(* Logix 5000 AddOnInstructionDefinition export Banner_Q4X_Teach_v4; software revision 36.00 *)

TYPE Banner_IOL_Port_v4 :   // UDT that has all of the data items necessary to communicate with a specific Port on a IO-Link Master
STRUCT
   Port_Controlled : INT;   // Each bit represents a port on an IO-Link Master. Set to 1 to tell AOI to control that port.
   Port_Activate : INT;   // Each bit represents a port on an IO-Link Master. When ON that port will process any commands in queue.
   Port_Read : INT;   // Each bit represents a port on an IO-Link Master. Used to determine when device AOI has requested a Read command.
   Port_Write : INT;   // Each bit represents a port on an IO-Link Master. Used to determine when device AOI has requested a Write command.
   Port_RW_Complete : INT;   // Each bit represents a port on an IO-Link Master. Tells device AOI that Read or Write request has been completed.
   Port_Device_Read : INT;
   Data_Transfer : SINT[190];   // Array to transfer data from IO-Master to device AOIs.
END_STRUCT
END_TYPE

TYPE Banner_Q4X_Data_v4 :   // UDT that stores Teach Data for a Q4X.
STRUCT
   System_Command : INT;   // Write Only. See IODD file for list of commands that can be activated via the System Command interface
   Teach_Channel : INT;   // RW. 0 = Default, 1 = BDC1, 2 = BDC2
   Teach_State : SINT;   // Read Only. 0 =IDLE, 1 = SP1 Success, 4 = Wait for Command, 5 = Busy, 7 = Error
   SP1_TP1 : SINT;   // Read Only. 0 = not taught or unsuccessful, 1 = successfully taught
   SP2_TP2 : SINT;   // Read Only. 0 = not taught or unsuccessful, 1 = successfully taught
   BDC1_Setpoint_SP1 : DINT;   // Switch point value in .1 mm increments. Range: varies depending on sensor.
   BDC1_Setpoint_SP2 : DINT;   // In FGS mode defines second switching point parameter. Range: varies depending on sensor.
   BDC2_Setpoint_SP1 : DINT;   // Switch point value in .1 mm increments. Range: varies depending on sensor.
   BDC2_Setpoint_SP2 : DINT;   // In FGS mode defines second switching point parameter. Range: varies depending on sensor.
END_STRUCT
END_TYPE

TYPE Banner_Q4X_v4 :   // All of the parameters for a Q4X.
STRUCT
   Initial_Global_Read : BOOL;   // Determines if all of the IO-Link data has been read into the PLC yet
   Command : INT;   // Value placed in here will activate a read or write to a specifc IO-Link Index
   Data : Banner_Q4X_Data_v4;   // Write Data
   Reset : BOOL;   // Resets AOI. This will force a complete parameter read of the sensor.
END_STRUCT
END_TYPE

ADD_ON_INSTRUCTION Banner_Q4X_Teach_v4   (* revision 4.2, vendor Banner Engineering *)
// AOI to read and write parameter data to an IO-Link Q4X.
// Revision note:
// AOI to only access Standard Command IO-Link function. This is used to teach the sensor. It also accesses the Teach Status.
VAR_IN_OUT
   Q4X : Banner_Q4X_v4; {required}
   Port_Data : Banner_IOL_Port_v4; {required}
END_VAR
VAR_INPUT
   Port : INT; {required}   // Enter the Port number that this AOI is to work with.
END_VAR
VAR_IN_OUT
   Teach : BOOL; {required}
END_VAR
VAR_OUTPUT
   Teach_Error : BOOL; {visible}
END_VAR
VAR
   Local_Control : DINT; {access None}
   Global_Read_Command_Value : INT; {access None}
   Global_Write_Command_Value : INT; {access None}
   Command_Being_Processed : BOOL; {access None}
   Update_Archive : BOOL; {access None}
   Index_Write_Inprocess : INT; {access None}
   Index_Write_Control : INT; {access None}
   Temp_Excess_Gain : DINT[2]; {access None}
   Inprocess_Index : DINT; {access None}
   Counter : COUNTER := (PRE := 20); {access None}
   WriteCheck : BOOL; {access None}
   Timer2 : TIMER := (PRE := 7500); {access None}
   Timer1 : TIMER := (PRE := 60000); {access None}
END_VAR

ROUTINE Logic   (* ladder *)
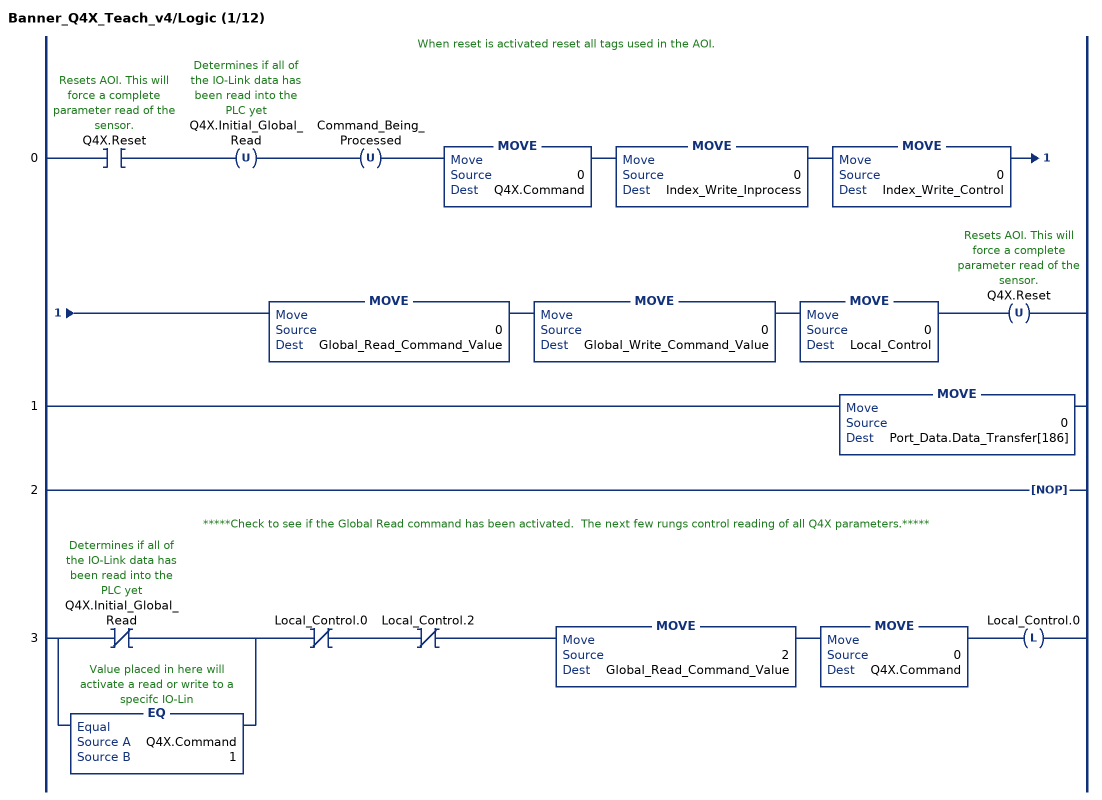
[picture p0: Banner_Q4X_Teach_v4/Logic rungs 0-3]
   // When reset is activated reset all tags used in the AOI.
   0: XIC(Q4X.Reset)OTU(Q4X.Initial_Global_Read)OTU(Command_Being_Processed)MOVE(0,Q4X.Command)MOVE(0,Index_Write_Inprocess)MOVE(0,Index_Write_Control)MOVE(0,Global_Read_Command_Value)MOVE(0,Global_Write_Command_Value)MOVE(0,Local_Control)OTU(Q4X.Reset);
   1: MOVE(0,Port_Data.Data_Transfer[186]);
   2: NOP();
   // *****Check to see if the Global Read command has been activated.  The next few rungs control reading of all Q4X parameters.*****
   3: [XIO(Q4X.Initial_Global_Read) ,EQ(Q4X.Command,1) ]XIO(Local_Control.0)XIO(Local_Control.2)MOVE(2,Global_Read_Command_Value)MOVE(0,Q4X.Command)OTL(Local_Control.0);
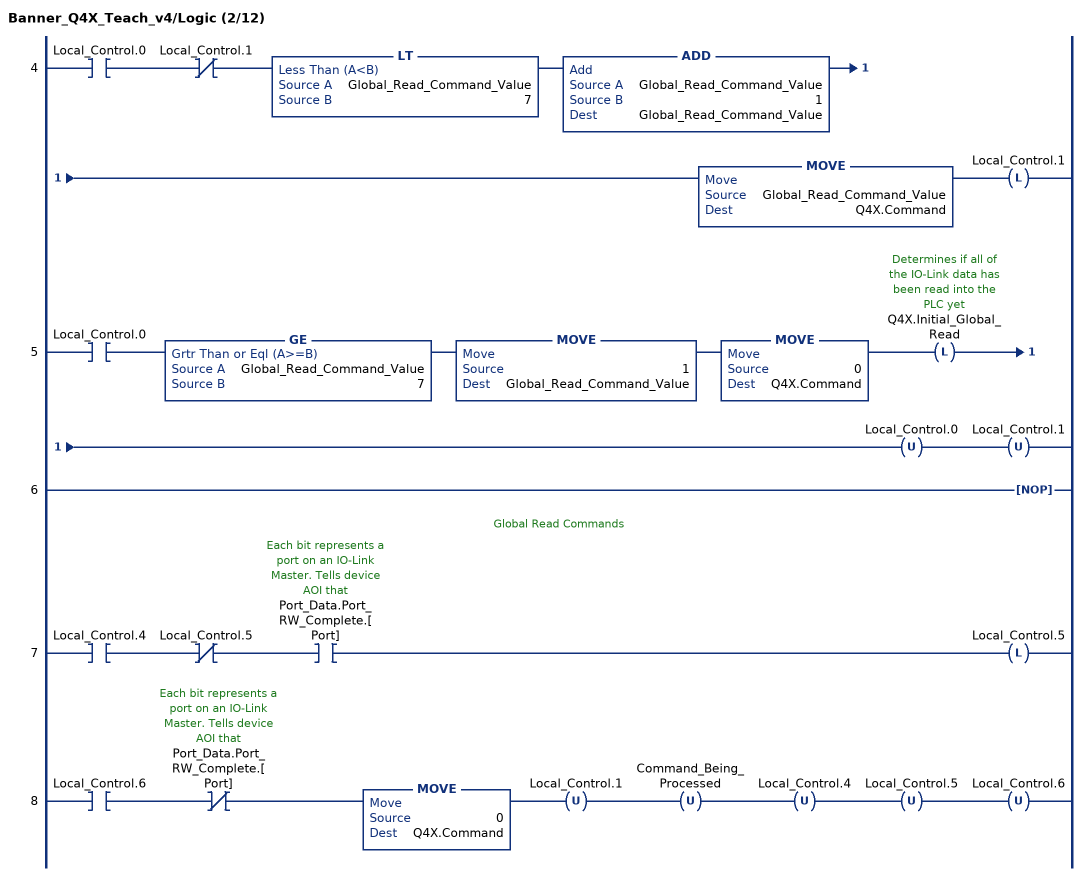
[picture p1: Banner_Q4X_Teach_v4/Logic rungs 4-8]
   4: XIC(Local_Control.0)XIO(Local_Control.1)LT(Global_Read_Command_Value,7)ADD(Global_Read_Command_Value,1,Global_Read_Command_Value)MOVE(Global_Read_Command_Value,Q4X.Command)OTL(Local_Control.1);
   5: XIC(Local_Control.0)GE(Global_Read_Command_Value,7)MOVE(1,Global_Read_Command_Value)MOVE(0,Q4X.Command)OTL(Q4X.Initial_Global_Read)OTU(Local_Control.0)OTU(Local_Control.1);
   6: NOP();
   // Global Read Commands
   7: XIC(Local_Control.4)XIO(Local_Control.5)XIC(Port_Data.Port_RW_Complete.[Port])OTL(Local_Control.5);
   8: XIC(Local_Control.6)XIO(Port_Data.Port_RW_Complete.[Port])MOVE(0,Q4X.Command)OTU(Local_Control.1)OTU(Command_Being_Processed)OTU(Local_Control.4)OTU(Local_Control.5)OTU(Local_Control.6);
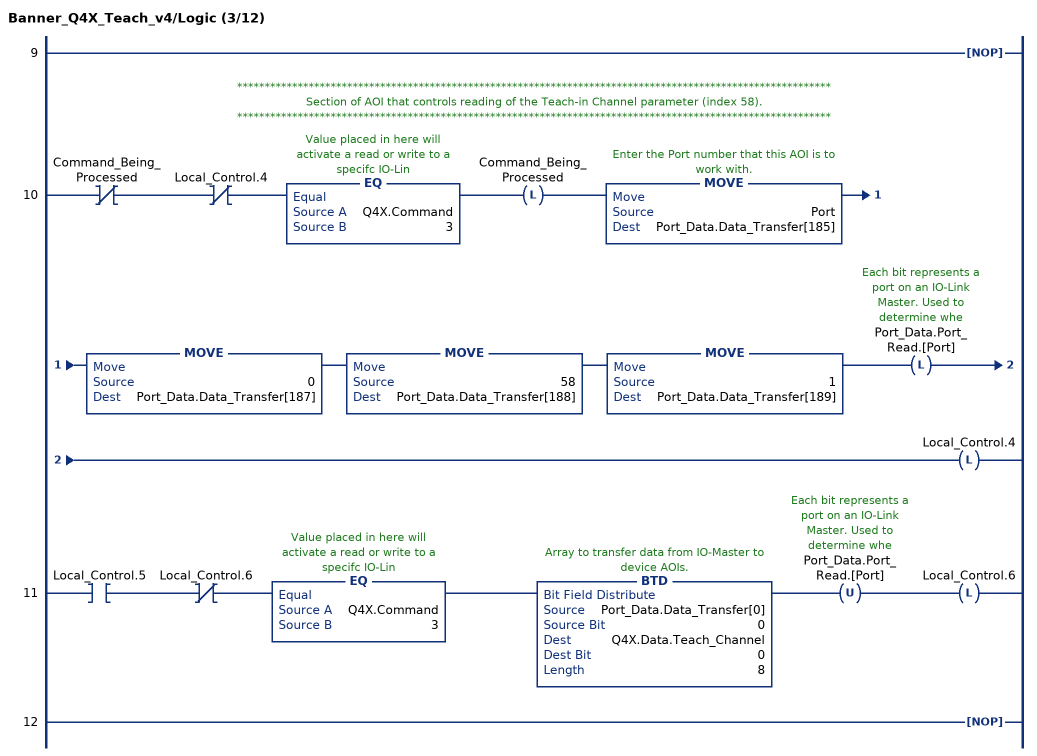
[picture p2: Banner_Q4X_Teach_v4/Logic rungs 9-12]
   9: NOP();
   // ************************************************************************************************************
   // Section of AOI that controls reading of the Teach-in Channel parameter (index 58).
   // ************************************************************************************************************
   10: XIO(Command_Being_Processed)XIO(Local_Control.4)EQ(Q4X.Command,3)OTL(Command_Being_Processed)MOVE(Port,Port_Data.Data_Transfer[185])MOVE(0,Port_Data.Data_Transfer[187])MOVE(58,Port_Data.Data_Transfer[188])MOVE(1,Port_Data.Data_Transfer[189])OTL(Port_Data.Port_Read.[Port])OTL(Local_Control.4);
   11: XIC(Local_Control.5)XIO(Local_Control.6)EQ(Q4X.Command,3)BTD(Port_Data.Data_Transfer[0],0,Q4X.Data.Teach_Channel,0,8)OTU(Port_Data.Port_Read.[Port])OTL(Local_Control.6);
   12: NOP();
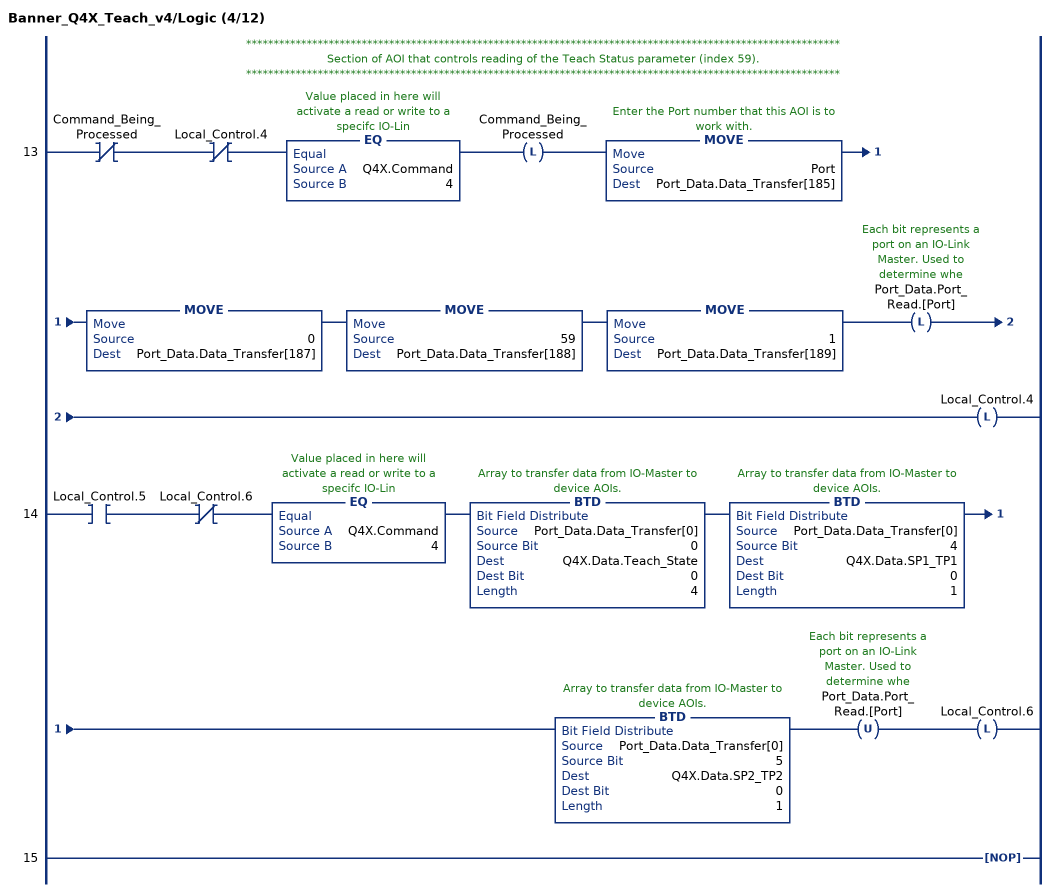
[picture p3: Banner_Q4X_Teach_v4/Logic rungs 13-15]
   // ************************************************************************************************************
   // Section of AOI that controls reading of the Teach Status parameter (index 59).
   // ************************************************************************************************************
   13: XIO(Command_Being_Processed)XIO(Local_Control.4)EQ(Q4X.Command,4)OTL(Command_Being_Processed)MOVE(Port,Port_Data.Data_Transfer[185])MOVE(0,Port_Data.Data_Transfer[187])MOVE(59,Port_Data.Data_Transfer[188])MOVE(1,Port_Data.Data_Transfer[189])OTL(Port_Data.Port_Read.[Port])OTL(Local_Control.4);
   14: XIC(Local_Control.5)XIO(Local_Control.6)EQ(Q4X.Command,4)BTD(Port_Data.Data_Transfer[0],0,Q4X.Data.Teach_State,0,4)BTD(Port_Data.Data_Transfer[0],4,Q4X.Data.SP1_TP1,0,1)BTD(Port_Data.Data_Transfer[0],5,Q4X.Data.SP2_TP2,0,1)OTU(Port_Data.Port_Read.[Port])OTL(Local_Control.6);
   15: NOP();
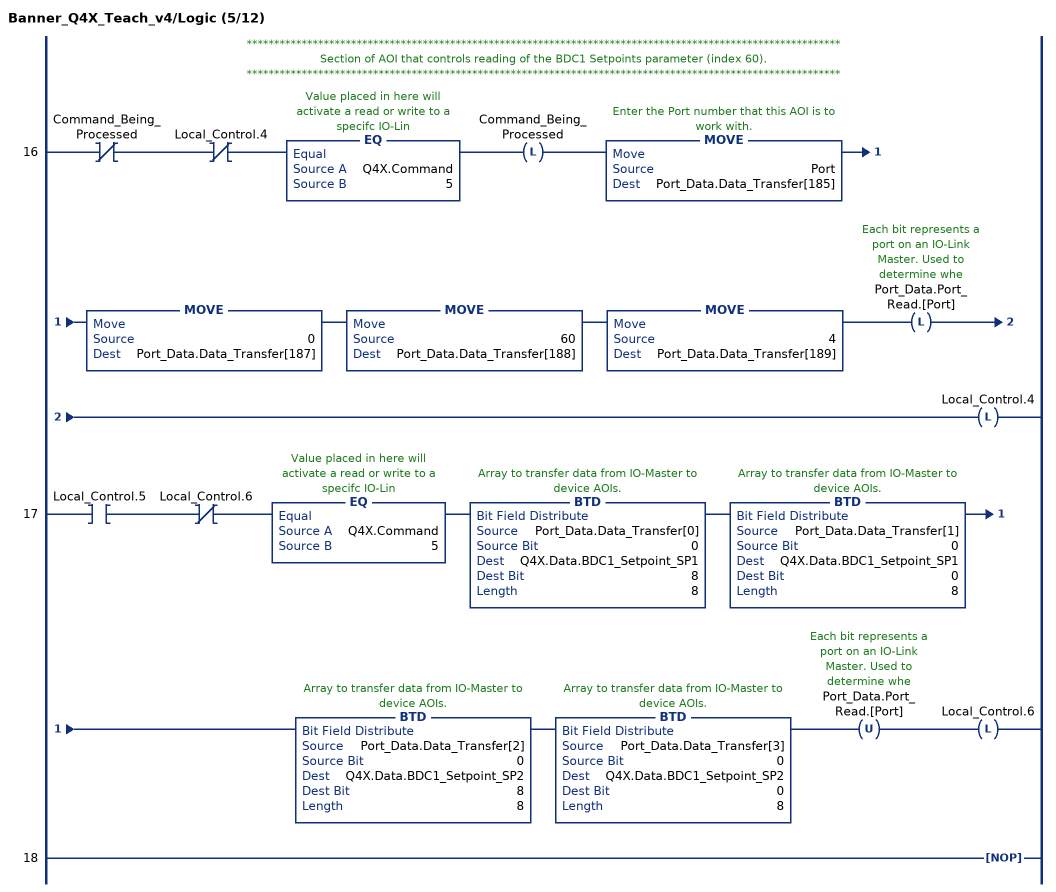
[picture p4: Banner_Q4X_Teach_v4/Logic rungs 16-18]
   // ************************************************************************************************************
   // Section of AOI that controls reading of the BDC1 Setpoints parameter (index 60).
   // ************************************************************************************************************
   16: XIO(Command_Being_Processed)XIO(Local_Control.4)EQ(Q4X.Command,5)OTL(Command_Being_Processed)MOVE(Port,Port_Data.Data_Transfer[185])MOVE(0,Port_Data.Data_Transfer[187])MOVE(60,Port_Data.Data_Transfer[188])MOVE(4,Port_Data.Data_Transfer[189])OTL(Port_Data.Port_Read.[Port])OTL(Local_Control.4);
   17: XIC(Local_Control.5)XIO(Local_Control.6)EQ(Q4X.Command,5)BTD(Port_Data.Data_Transfer[0],0,Q4X.Data.BDC1_Setpoint_SP1,8,8)BTD(Port_Data.Data_Transfer[1],0,Q4X.Data.BDC1_Setpoint_SP1,0,8)BTD(Port_Data.Data_Transfer[2],0,Q4X.Data.BDC1_Setpoint_SP2,8,8)BTD(Port_Data.Data_Transfer[3],0,Q4X.Data.BDC1_Setpoint_SP2,0,8)OTU(Port_Data.Port_Read.[Port])OTL(Local_Control.6);
   18: NOP();
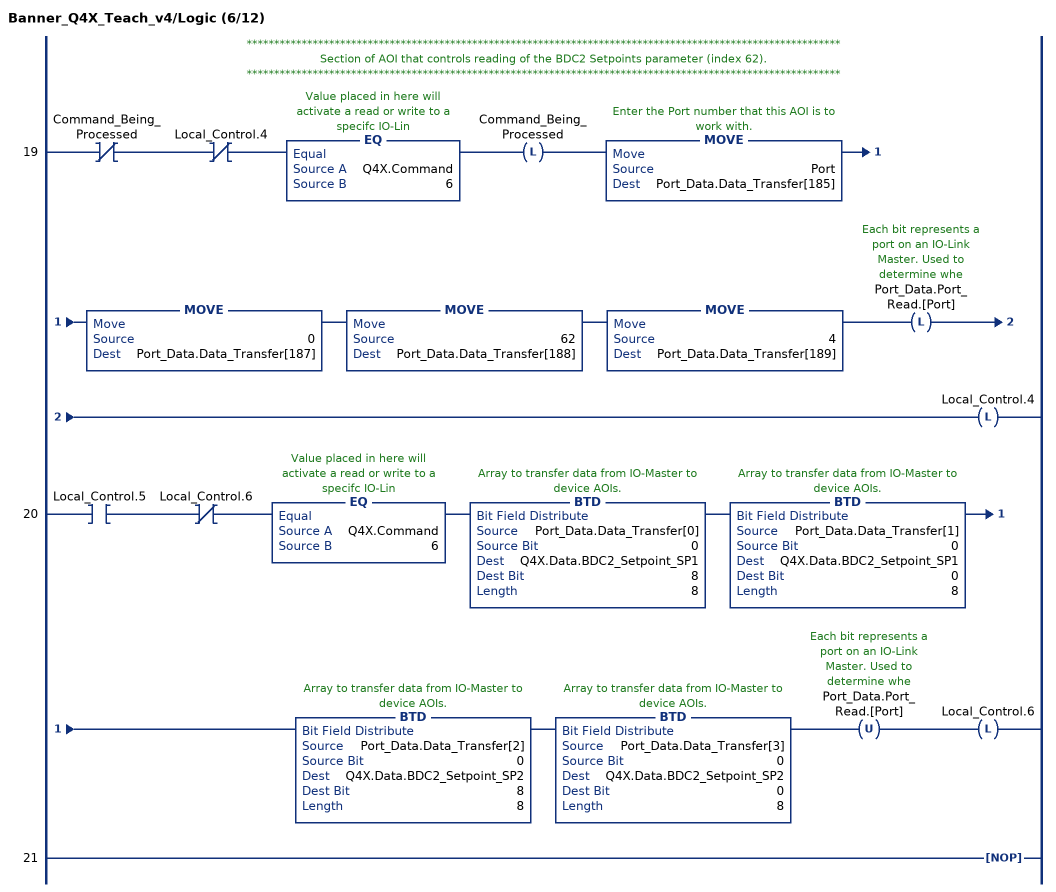
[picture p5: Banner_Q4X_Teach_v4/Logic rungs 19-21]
   // ************************************************************************************************************
   // Section of AOI that controls reading of the BDC2 Setpoints parameter (index 62).
   // ************************************************************************************************************
   19: XIO(Command_Being_Processed)XIO(Local_Control.4)EQ(Q4X.Command,6)OTL(Command_Being_Processed)MOVE(Port,Port_Data.Data_Transfer[185])MOVE(0,Port_Data.Data_Transfer[187])MOVE(62,Port_Data.Data_Transfer[188])MOVE(4,Port_Data.Data_Transfer[189])OTL(Port_Data.Port_Read.[Port])OTL(Local_Control.4);
   20: XIC(Local_Control.5)XIO(Local_Control.6)EQ(Q4X.Command,6)BTD(Port_Data.Data_Transfer[0],0,Q4X.Data.BDC2_Setpoint_SP1,8,8)BTD(Port_Data.Data_Transfer[1],0,Q4X.Data.BDC2_Setpoint_SP1,0,8)BTD(Port_Data.Data_Transfer[2],0,Q4X.Data.BDC2_Setpoint_SP2,8,8)BTD(Port_Data.Data_Transfer[3],0,Q4X.Data.BDC2_Setpoint_SP2,0,8)OTU(Port_Data.Port_Read.[Port])OTL(Local_Control.6);
   21: NOP();
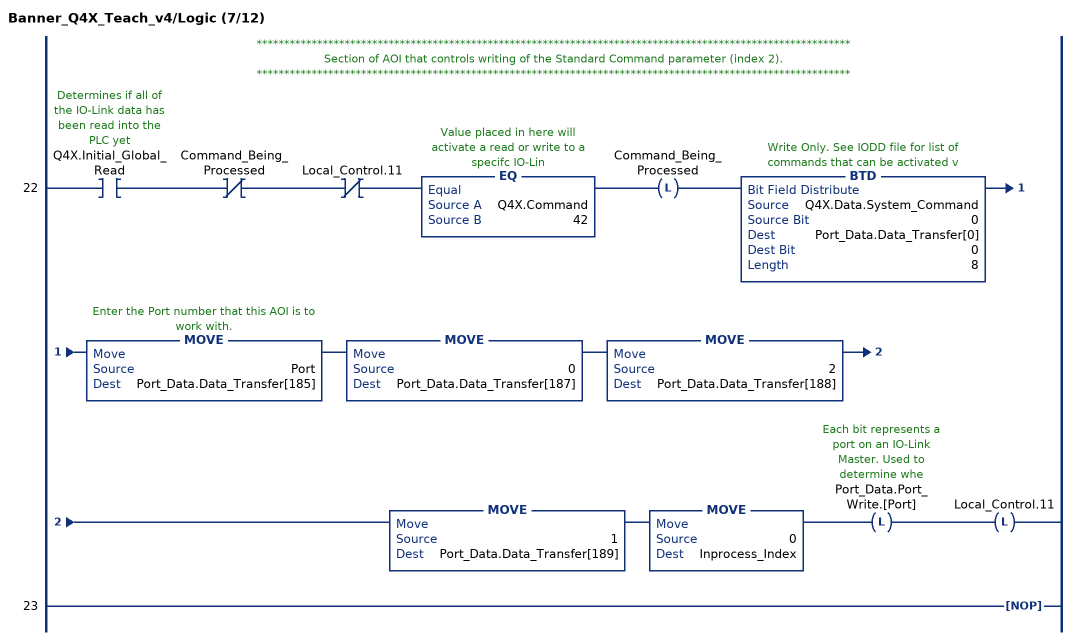
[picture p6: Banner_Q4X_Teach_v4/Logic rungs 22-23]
   // ************************************************************************************************************
   // Section of AOI that controls writing of the Standard Command parameter (index 2).
   // ************************************************************************************************************
   22: XIC(Q4X.Initial_Global_Read)XIO(Command_Being_Processed)XIO(Local_Control.11)EQ(Q4X.Command,42)OTL(Command_Being_Processed)BTD(Q4X.Data.System_Command,0,Port_Data.Data_Transfer[0],0,8)MOVE(Port,Port_Data.Data_Transfer[185])MOVE(0,Port_Data.Data_Transfer[187])MOVE(2,Port_Data.Data_Transfer[188])MOVE(1,Port_Data.Data_Transfer[189])MOVE(0,Inprocess_Index)OTL(Port_Data.Port_Write.[Port])OTL(Local_Control.11);
   23: NOP();
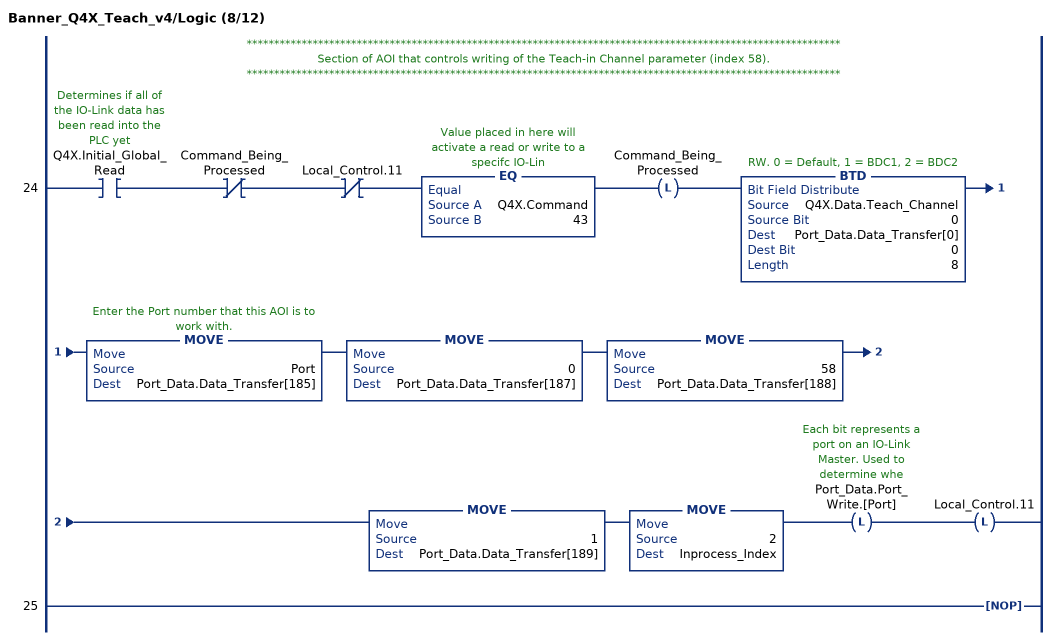
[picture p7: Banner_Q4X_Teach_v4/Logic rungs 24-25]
   // ************************************************************************************************************
   // Section of AOI that controls writing of the Teach-in Channel parameter (index 58).
   // ************************************************************************************************************
   24: XIC(Q4X.Initial_Global_Read)XIO(Command_Being_Processed)XIO(Local_Control.11)EQ(Q4X.Command,43)OTL(Command_Being_Processed)BTD(Q4X.Data.Teach_Channel,0,Port_Data.Data_Transfer[0],0,8)MOVE(Port,Port_Data.Data_Transfer[185])MOVE(0,Port_Data.Data_Transfer[187])MOVE(58,Port_Data.Data_Transfer[188])MOVE(1,Port_Data.Data_Transfer[189])MOVE(2,Inprocess_Index)OTL(Port_Data.Port_Write.[Port])OTL(Local_Control.11);
   25: NOP();
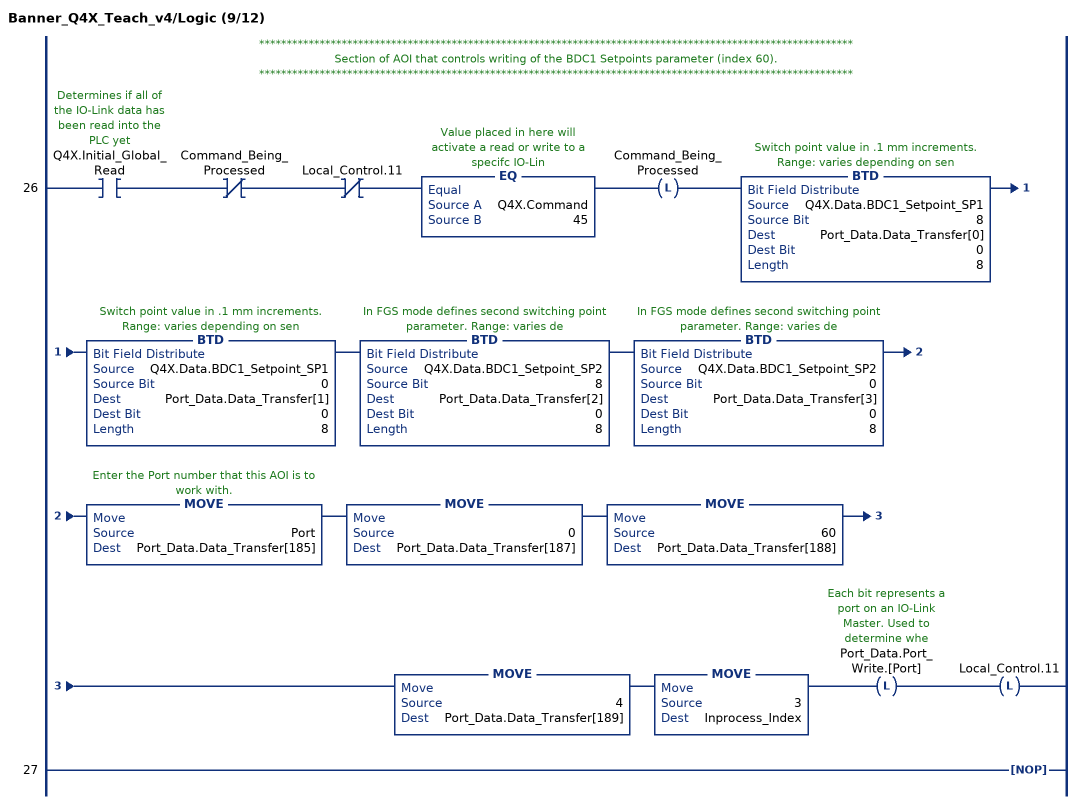
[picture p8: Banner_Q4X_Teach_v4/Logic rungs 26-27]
   // ************************************************************************************************************
   // Section of AOI that controls writing of the BDC1 Setpoints parameter (index 60).
   // ************************************************************************************************************
   26: XIC(Q4X.Initial_Global_Read)XIO(Command_Being_Processed)XIO(Local_Control.11)EQ(Q4X.Command,45)OTL(Command_Being_Processed)BTD(Q4X.Data.BDC1_Setpoint_SP1,8,Port_Data.Data_Transfer[0],0,8)BTD(Q4X.Data.BDC1_Setpoint_SP1,0,Port_Data.Data_Transfer[1],0,8)BTD(Q4X.Data.BDC1_Setpoint_SP2,8,Port_Data.Data_Transfer[2],0,8)BTD(Q4X.Data.BDC1_Setpoint_SP2,0,Port_Data.Data_Transfer[3],0,8)MOVE(Port,Port_Data.Data_Transfer[185])MOVE(0,Port_Data.Data_Transfer[187])MOVE(60,Port_Data.Data_Transfer[188])MOVE(4,Port_Data.Data_Transfer[189])MOVE(3,Inprocess_Index)OTL(Port_Data.Port_Write.[Port])OTL(Local_Control.11);
   27: NOP();
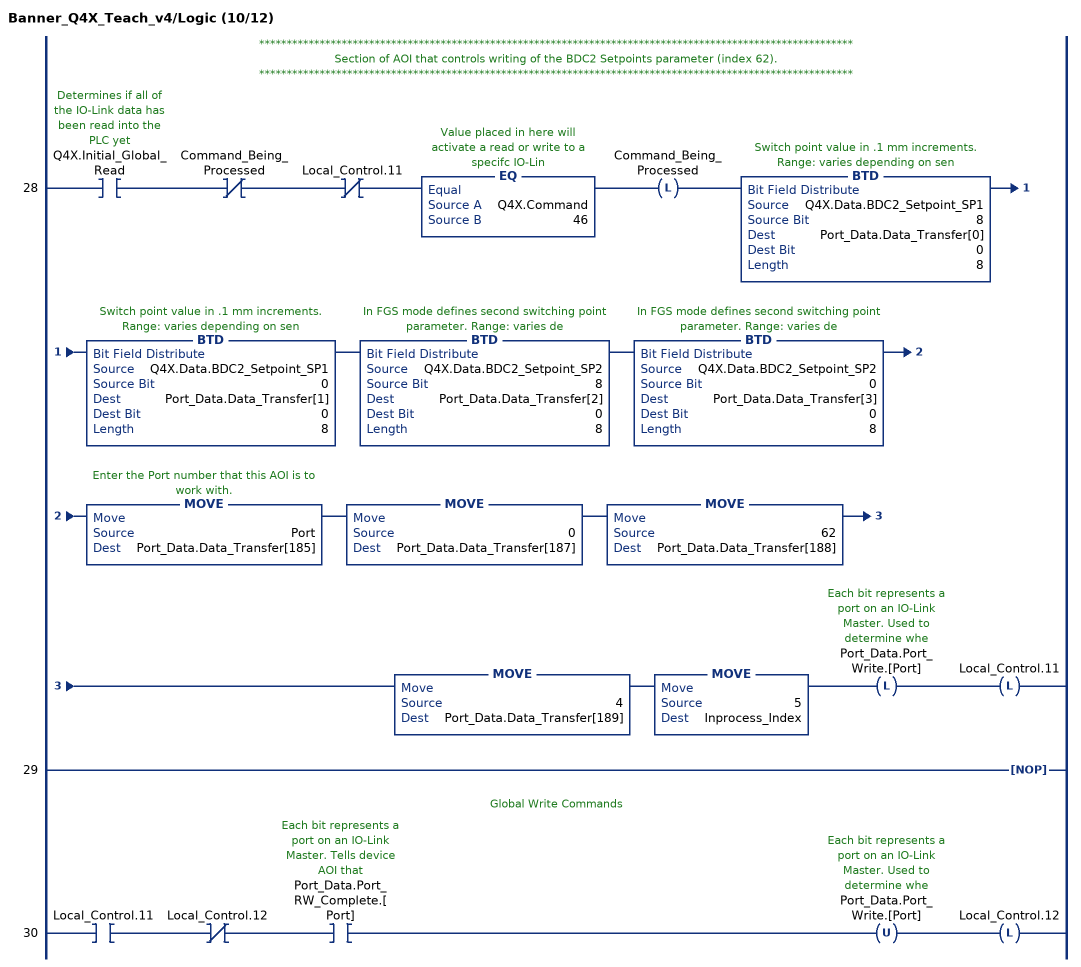
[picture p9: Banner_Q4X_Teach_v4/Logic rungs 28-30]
   // ************************************************************************************************************
   // Section of AOI that controls writing of the BDC2 Setpoints parameter (index 62).
   // ************************************************************************************************************
   28: XIC(Q4X.Initial_Global_Read)XIO(Command_Being_Processed)XIO(Local_Control.11)EQ(Q4X.Command,46)OTL(Command_Being_Processed)BTD(Q4X.Data.BDC2_Setpoint_SP1,8,Port_Data.Data_Transfer[0],0,8)BTD(Q4X.Data.BDC2_Setpoint_SP1,0,Port_Data.Data_Transfer[1],0,8)BTD(Q4X.Data.BDC2_Setpoint_SP2,8,Port_Data.Data_Transfer[2],0,8)BTD(Q4X.Data.BDC2_Setpoint_SP2,0,Port_Data.Data_Transfer[3],0,8)MOVE(Port,Port_Data.Data_Transfer[185])MOVE(0,Port_Data.Data_Transfer[187])MOVE(62,Port_Data.Data_Transfer[188])MOVE(4,Port_Data.Data_Transfer[189])MOVE(5,Inprocess_Index)OTL(Port_Data.Port_Write.[Port])OTL(Local_Control.11);
   29: NOP();
   // Global Write Commands
   30: XIC(Local_Control.11)XIO(Local_Control.12)XIC(Port_Data.Port_RW_Complete.[Port])OTU(Port_Data.Port_Write.[Port])OTL(Local_Control.12);
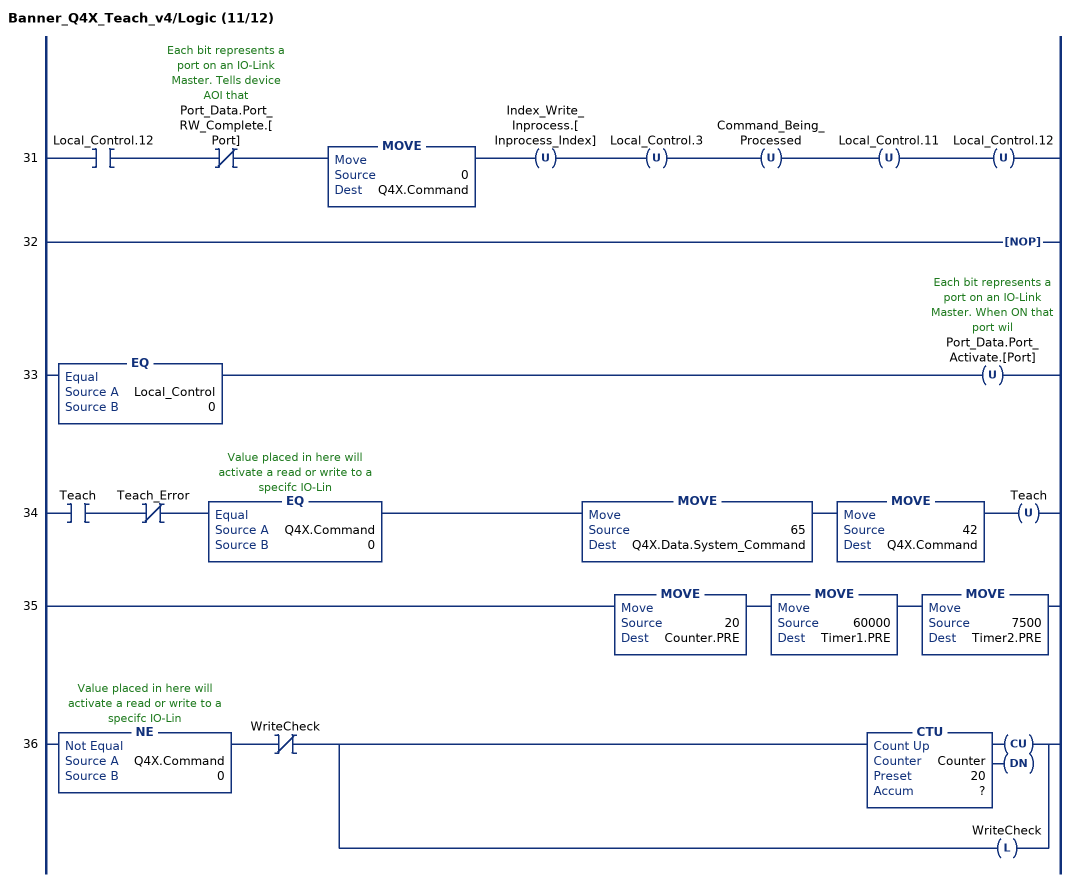
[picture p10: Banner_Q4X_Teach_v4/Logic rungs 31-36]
   31: XIC(Local_Control.12)XIO(Port_Data.Port_RW_Complete.[Port])MOVE(0,Q4X.Command)OTU(Index_Write_Inprocess.[Inprocess_Index])OTU(Local_Control.3)OTU(Command_Being_Processed)OTU(Local_Control.11)OTU(Local_Control.12);
   32: NOP();
   33: EQ(Local_Control,0)OTU(Port_Data.Port_Activate.[Port]);
   34: XIC(Teach)XIO(Teach_Error)EQ(Q4X.Command,0)MOVE(65,Q4X.Data.System_Command)MOVE(42,Q4X.Command)OTU(Teach);
   35: MOVE(20,Counter.PRE)MOVE(60000,Timer1.PRE)MOVE(7500,Timer2.PRE);
   36: NE(Q4X.Command,0)XIO(WriteCheck)[CTU(Counter,?,?) ,OTL(WriteCheck) ];
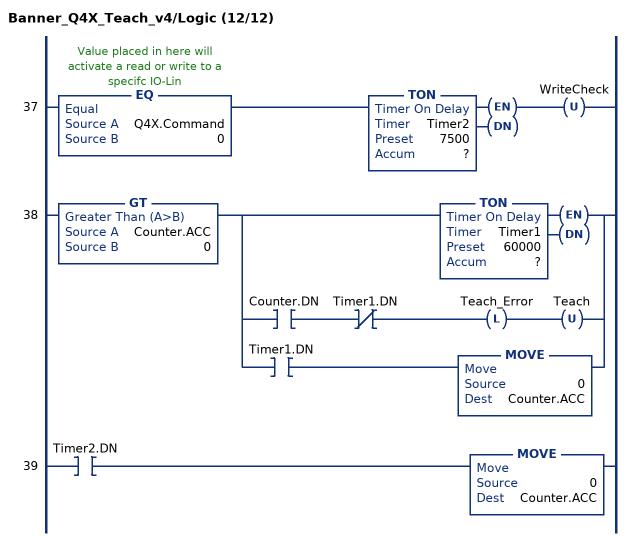
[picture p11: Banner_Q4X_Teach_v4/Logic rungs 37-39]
   37: EQ(Q4X.Command,0)TON(Timer2,?,?)OTU(WriteCheck);
   38: GT(Counter.ACC,0)[TON(Timer1,?,?) ,XIC(Counter.DN) XIO(Timer1.DN) OTL(Teach_Error) OTU(Teach) ,XIC(Timer1.DN) MOVE(0,Counter.ACC) ];
   39: XIC(Timer2.DN)MOVE(0,Counter.ACC);
END_ROUTINE
END_ADD_ON_INSTRUCTION
